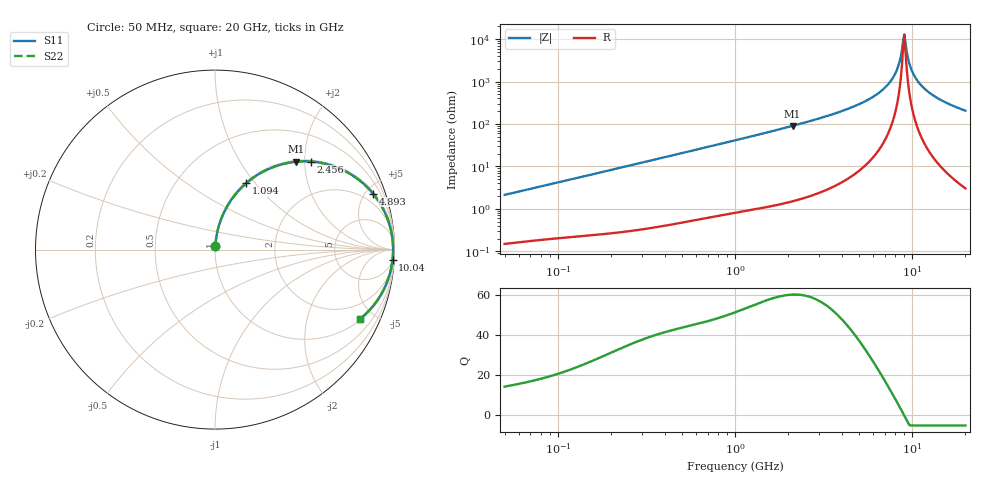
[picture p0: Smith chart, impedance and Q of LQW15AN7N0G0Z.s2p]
!Murata Part Number: LQW15AN7N0G0Z
!These Parameters are Measured in Series Mode Connection
!  o--[Z]--o
!Port1  Port2
!  o-------o
!Freq. Start=50[MHz] Stop=20[GHz], 401[Steps]
# Hz S RI R 50
!Freq.(Hz) S11(Real) S11(Imag) S21(Real) S21(Imag) S12(Real) S12(Imag) S22(Real) S22(Imag)
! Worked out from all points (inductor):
!   401 points, 50 MHz to 20 GHz, reference 50 ohm
!   read as one part in series: L = 6.74 nH near 51.52 MHz
!   highest Q = 60.1 at 2.115 GHz (marker M1), where L = 6.81 nH
!   self-resonance near 8.907 GHz
!   S11 on the Smith chart (normalised r, x): 50 MHz: 1.00, +0.04; 1.094 GHz: 1.02, +0.90; 2.456 GHz: 1.04, +2.15; 4.893 GHz: 1.15, +5.59; 10.04 GHz: 5, -34; 20 GHz: 1.06, -4.13
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5e7  0.00194 0.0212  0.9981 -0.0212  0.9981 -0.0212  0.00194 0.0212
1.364002e8  0.00546 0.0564  0.9945 -0.0564  0.9945 -0.0564  0.00546 0.0564
3.721004e8  0.0265 0.1488  0.9735 -0.1488  0.9735 -0.1488  0.0265 0.1488
1e9  0.15 0.3474  0.85 -0.3474  0.85 -0.3474  0.15 0.3474
1.094034e9  0.174 0.3697  0.826 -0.3697  0.826 -0.3697  0.174 0.3697
2.114743e9  0.4513 0.4894  0.5487 -0.4894  0.5487 -0.4894  0.4513 0.4894
2.456456e9  0.5346 0.4905  0.4654 -0.4905  0.4654 -0.4905  0.5346 0.4905
2.728004e9  0.5941 0.4826  0.4059 -0.4826  0.4059 -0.4826  0.5941 0.4826
4.89267e9  0.8805 0.3117  0.1195 -0.3117  0.1195 -0.3117  0.8805 0.3117
6.311513e9  0.954 0.1897  0.046 -0.1897  0.046 -0.1897  0.954 0.1897
7.442007e9  0.9811 0.1037  0.0189 -0.1037  0.0189 -0.1037  0.9811 0.1037
8.264682e9  0.99 0.0475  0.01 -0.0475  0.01 -0.0475  0.99 0.0475
8.516016e9  0.9913 0.0314  0.00869 -0.0314  0.00869 -0.0314  0.9913 0.0314
8.774992e9  0.9921 0.0152  0.00789 -0.0152  0.00789 -0.0152  0.9921 0.0152
9.041845e9  0.9924 -0.000993  0.00761 0.000993  0.00761 0.000993  0.9924 -0.000993
9.178299e9  0.9923 -0.00909  0.00768 0.00909  0.00768 0.00909  0.9923 -0.00909
9.600142e9  0.9913 -0.0334  0.00866 0.0334  0.00866 0.0334  0.9913 -0.0334
1.004137e10  0.9892 -0.0576  0.0108 0.0576  0.0108 0.0576  0.9892 -0.0576
1.098561e10  0.9812 -0.1058  0.0188 0.1058  0.0188 0.1058  0.9812 -0.1058
1.276073e10  0.9572 -0.1843  0.0428 0.1843  0.0428 0.1843  0.9572 -0.1843
1.573793e10  0.9012 -0.2874  0.0988 0.2874  0.0988 0.2874  0.9012 -0.2874
2e10  0.8064 -0.3878  0.1936 0.3878  0.1936 0.3878  0.8064 -0.3878
